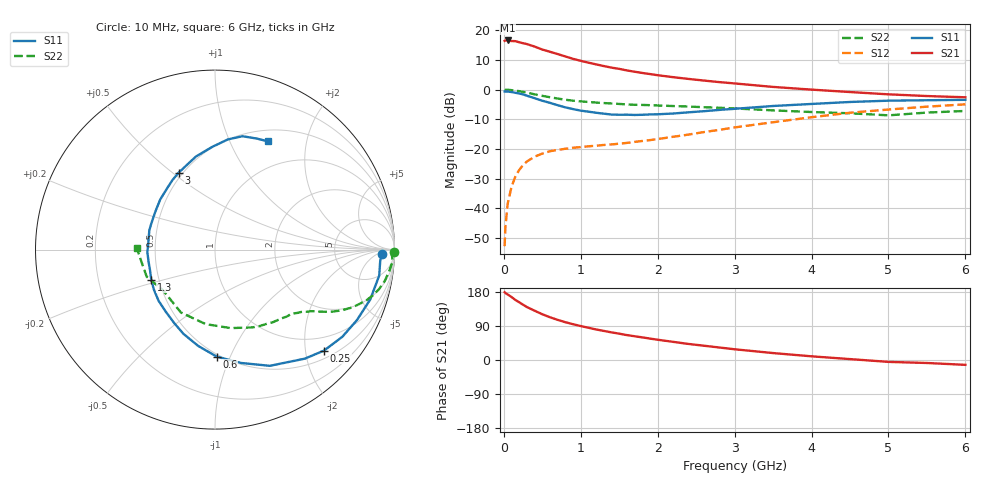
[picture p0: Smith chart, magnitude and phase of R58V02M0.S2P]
! SIEMENS Small Signal Semiconductors
! BFR183
! Si NPN RF Bipolar Junction Transistor in SOT23
! VCE = 8 V  IC = 2 mA
! Common Emitter S-Parameters:  May  1996
# GHz  S  MA  R  50
!  f  S11  S21  S12  S22
! GHz  MAG  ANG  MAG  ANG  MAG  ANG  MAG  ANG
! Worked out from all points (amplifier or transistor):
!   36 points, 10 MHz to 6 GHz, reference 50 ohm
!   highest |S21| = 16.5 dB at 50 MHz (marker M1)
!   |S21| within 3 dB of that: start of sweep to 493.1 MHz
!   unconditionally stable (mu >= 1): 1.437 GHz to 2.849 GHz
!   at 250 MHz: K = 0.22, MSG = 20.5 dB, |S12| = -25.4 dB
!   at 1.4 GHz: K = 0.99, MSG = 12.9 dB, |S12| = -18.5 dB
!   at 6 GHz: K = 0.89, MSG = 1.2 dB, |S12| = -5.0 dB
!   S11 on the Smith chart (normalised r, x): 10 MHz: 24, -9; 250 MHz: 0.67, -2.39; 600 MHz: 0.48, -0.89; 1.3 GHz: 0.45, -0.18; 3 GHz: 0.48, +0.53; 6 GHz: 0.64, +1.40
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0.01  0.9298 -1.6  6.607 178.8  0.0023 89.5  0.9958 -0.7
0.02  0.9226 -3.9  6.719 176.9  0.0048 85.8  0.9847 -1.4
0.05  0.9263 -9.0  6.719 172.9  0.0119 85.2  0.9923 -3.7
0.1  0.9084 -17.8  6.566 166.2  0.0231 80.0  0.978 -7.1
0.15  0.8831 -26.4  6.541 158.4  0.0342 74.6  0.9611 -10.6
0.25  0.828 -42.8  6.033 145.9  0.0534 66.3  0.9153 -16.2
0.3  0.7873 -50.5  5.843 139.7  0.0615 63.0  0.8876 -18.7
0.4  0.7162 -64.7  5.299 130.1  0.074 56.9  0.8307 -22.8
0.5  0.6483 -77.0  4.719 120.7  0.0835 52.1  0.7832 -25.6
0.6  0.5968 -89.0  4.332 112.8  0.0914 48.7  0.7427 -27.7
0.7  0.5448 -99.9  3.965 105.9  0.0962 46.3  0.7058 -29.4
0.8  0.5013 -110.5  3.61 99.7  0.1007 44.6  0.6739 -30.8
0.9  0.4687 -118.9  3.292 94.4  0.1046 44.0  0.6498 -31.9
1.1  0.4245 -137.8  2.84 85.1  0.1106 43.0  0.6178 -34.1
1.3  0.3925 -154.8  2.487 76.7  0.1166 43.9  0.5924 -35.9
1.6  0.3771 -177.9  2.099 65.7  0.1263 46.8  0.5624 -39.3
2.2  0.3948 147.0  1.618 47.9  0.1601 52.8  0.5277 -47.7
3  0.474 115.3  1.268 28.3  0.2303 54.1  0.481 -64.3
3.5  0.5288 101.7  1.108 18.3  0.2818 50.9  0.446 -78.7
4.5  0.6177 83.4  0.908 2.4  0.4074 40.1  0.3985 -118.5
5.5  0.661 69.4  0.778 -7.9  0.5153 25.7  0.4095 -158.4
6  0.6716 63.8  0.741 -12.8  0.5637 16.7  0.4363 178.9
